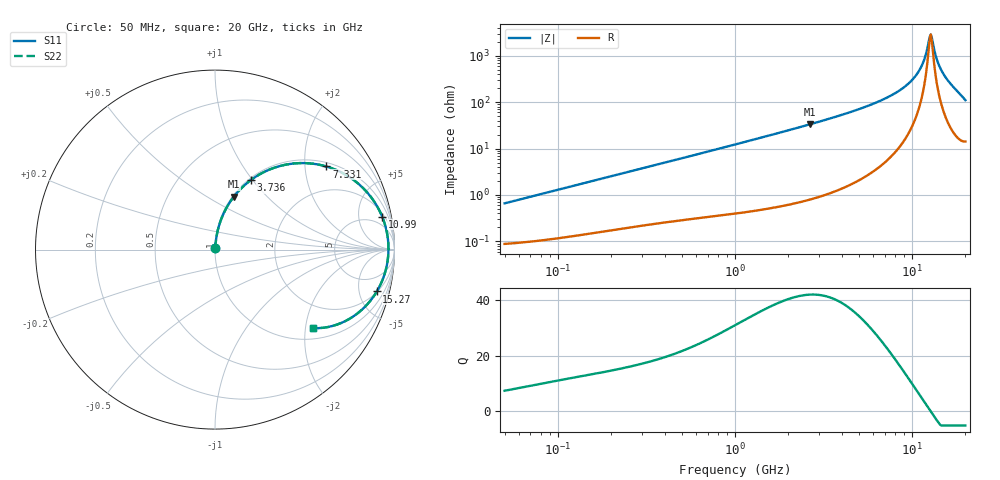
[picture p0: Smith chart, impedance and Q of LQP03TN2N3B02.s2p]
!Murata Part Number: LQP03TN2N3B02
!These Parameters are Measured in Series Mode Connection
!  o--[Z]--o
!Port1  Port2
!  o-------o
!Freq. Start=50[MHz] Stop=20[GHz], 401[Steps]
# Hz S RI R 50
!Freq.(Hz) S11(Real) S11(Imag) S21(Real) S21(Imag) S12(Real) S12(Imag) S22(Real) S22(Imag)
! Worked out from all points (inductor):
!   401 points, 50 MHz to 20 GHz, reference 50 ohm
!   read as one part in series: L = 2.08 nH near 51.52 MHz
!   highest Q = 41.8 at 2.647 GHz (marker M1), where L = 2 nH
!   self-resonance near 12.57 GHz
!   S11 on the Smith chart (normalised r, x): 50 MHz: 1.00, +0.01; 3.736 GHz: 1.02, +0.98; 7.331 GHz: 1.12, +2.58; 10.99 GHz: 2.58, +9.57; 15.27 GHz: 2.07, -7.27; 20 GHz: 1.28, -2.19
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5e7  0.000924 0.00654  0.9991 -0.00654  0.9991 -0.00654  0.000924 0.00654
1.364002e8  0.00168 0.0174  0.9983 -0.0174  0.9983 -0.0174  0.00168 0.0174
3.721004e8  0.00457 0.0459  0.9954 -0.0459  0.9954 -0.0459  0.00457 0.0459
1e9  0.0185 0.1195  0.9815 -0.1195  0.9815 -0.1195  0.0185 0.1195
2.647493e9  0.1054 0.2953  0.8946 -0.2953  0.8946 -0.2953  0.1054 0.2953
2.728004e9  0.1114 0.3029  0.8886 -0.3029  0.8886 -0.3029  0.1114 0.3029
3.736399e9  0.1995 0.3873  0.8005 -0.3873  0.8005 -0.3873  0.1995 0.3873
5.194772e9  0.3595 0.465  0.6405 -0.465  0.6405 -0.465  0.3595 0.465
7.331367e9  0.6204 0.4632  0.3796 -0.4632  0.3796 -0.4632  0.6204 0.4632
7.442007e9  0.6334 0.4592  0.3666 -0.4592  0.3666 -0.4592  0.6334 0.4592
9.457416e9  0.8372 0.3304  0.1628 -0.3304  0.1628 -0.3304  0.8372 0.3304
1.034674e10  0.8994 0.248  0.1006 -0.248  0.1006 -0.248  0.8994 0.248
1.098561e10  0.9315 0.1833  0.0685 -0.1833  0.0685 -0.1833  0.9315 0.1833
1.166392e10  0.9541 0.1123  0.0459 -0.1123  0.0459 -0.1123  0.9541 0.1123
1.238412e10  0.9654 0.0366  0.0346 -0.0366  0.0346 -0.0366  0.9654 0.0366
1.276073e10  0.9665 -0.00238  0.0335 0.00238  0.0335 0.00238  0.9665 -0.00238
1.314879e10  0.9642 -0.0417  0.0358 0.0417  0.0358 0.0417  0.9642 -0.0417
1.375312e10  0.9546 -0.1008  0.0454 0.1008  0.0454 0.1008  0.9546 -0.1008
1.417136e10  0.9438 -0.1398  0.0562 0.1398  0.0562 0.1398  0.9438 -0.1398
1.527346e10  0.9014 -0.2333  0.0986 0.2333  0.0986 0.2333  0.9014 -0.2333
1.721783e10  0.7867 -0.3609  0.2133 0.3609  0.2133 0.3609  0.7867 -0.3609
2e10  0.5432 -0.4375  0.4568 0.4375  0.4568 0.4375  0.5432 -0.4375
